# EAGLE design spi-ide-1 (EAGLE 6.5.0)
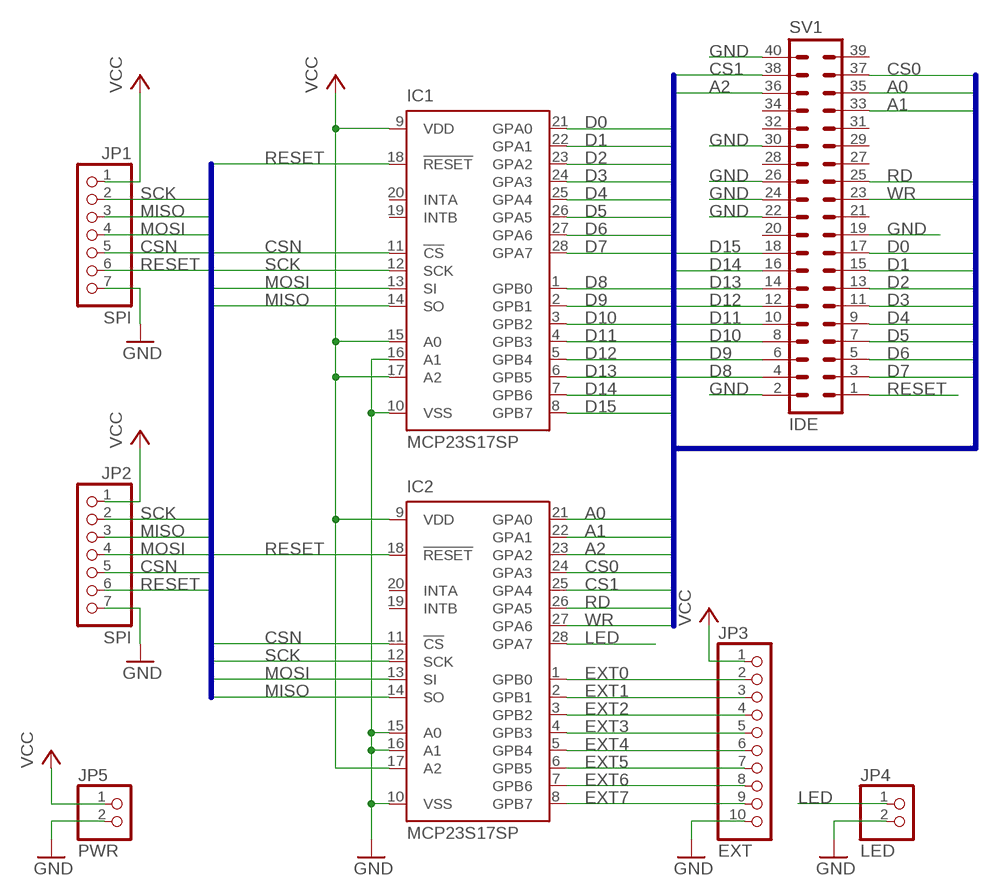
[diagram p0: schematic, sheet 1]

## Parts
IC1  MCP23S17SP  [DIL28-3]
IC2  MCP23S17SP  [DIL28-3]
JP1  SPI  PINHD-1X7  [1X07]
JP2  SPI  PINHD-1X7  [1X07]
JP3  EXT  PINHD-1X10  [1X10]
JP4  LED  PINHD-1X2  [1X02]
JP5  PWR  PINHD-1X2  [1X02]
SV1  IDE  ML40L  [ML40L]

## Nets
A0: IC2.21(GPA0) SV1.35
A1: IC2.22(GPA1) SV1.33
A2: IC2.23(GPA2) SV1.36
CS0: IC2.24(GPA3) SV1.37
CS1: IC2.25(GPA4) SV1.38
CSN: IC1.11(!CS) IC2.11(!CS) JP1.5 JP2.5
D0: IC1.21(GPA0) SV1.17
D1: IC1.22(GPA1) SV1.15
D2: IC1.23(GPA2) SV1.13
D3: IC1.24(GPA3) SV1.11
D4: IC1.25(GPA4) SV1.9
D5: IC1.26(GPA5) SV1.7
D6: IC1.27(GPA6) SV1.5
D7: IC1.28(GPA7) SV1.3
D8: IC1.1(GPB0) SV1.4
D9: IC1.2(GPB1) SV1.6
D10: IC1.3(GPB2) SV1.8
D11: IC1.4(GPB3) SV1.10
D12: IC1.5(GPB4) SV1.12
D13: IC1.6(GPB5) SV1.14
D14: IC1.7(GPB6) SV1.16
D15: IC1.8(GPB7) SV1.18
EXT0: IC2.1(GPB0) JP3.2
EXT1: IC2.2(GPB1) JP3.3
EXT2: IC2.3(GPB2) JP3.4
EXT3: IC2.4(GPB3) JP3.5
EXT4: IC2.5(GPB4) JP3.6
EXT5: IC2.6(GPB5) JP3.7
EXT6: IC2.7(GPB6) JP3.8
EXT7: IC2.8(GPB7) JP3.9
GND: IC1.10(VSS) IC1.16(A1) IC2.10(VSS) IC2.15(A0) IC2.16(A1) JP1.7 JP2.7 JP3.10 JP4.2 JP5.2 SV1.2 SV1.19 SV1.22 SV1.24 SV1.26 SV1.30 SV1.40
LED: IC2.28(GPA7) JP4.1
MISO: IC1.14(SO) IC2.14(SO) JP1.3 JP2.3
MOSI: IC1.13(SI) IC2.13(SI) JP1.4 JP2.4
RD: IC2.26(GPA5) SV1.25
RESET: IC1.18(!RESET) IC2.18(!RESET) JP1.6 JP2.6 SV1.1
SCK: IC1.12(SCK) IC2.12(SCK) JP1.2 JP2.2
VCC: IC1.9(VDD) IC1.15(A0) IC1.17(A2) IC2.9(VDD) IC2.17(A2) JP1.1 JP2.1 JP3.1 JP5.1
WR: IC2.27(GPA6) SV1.23
Unconnected: IC1.19(INTB) IC1.20(INTA) IC2.19(INTB) IC2.20(INTA) SV1.20 SV1.21 SV1.27 SV1.28 SV1.29 SV1.31 SV1.32 SV1.34 SV1.39

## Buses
BUS_SPI:SCK,MISO,MOSI,CSN,RESET
IDE:D[0..15],A[0..2],CS[0..1],RD,WR

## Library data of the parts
IC1 IC2 = microchip:MCP23S17: http://ww1.microchip.com/downloads/en/DeviceDoc/21952a.pdf Source: http://ww1.microchip.com/downloads/en/DeviceDoc/21952a.pdf; MF: MICROCHIP; MPN: MCP23S17-E/SP; OC_FARNELL: 1292238; OC_NEWARK: 31K2951
JP1 JP2 = pinhead:PINHD-1X7: PIN HEADER
JP3 = pinhead:PINHD-1X10: PIN HEADER
JP4 JP5 = pinhead:PINHD-1X2: PIN HEADER
SV1 = con-harting-ml:ML40: HARTING; OC_FARNELL: unknown; OC_NEWARK: unknown

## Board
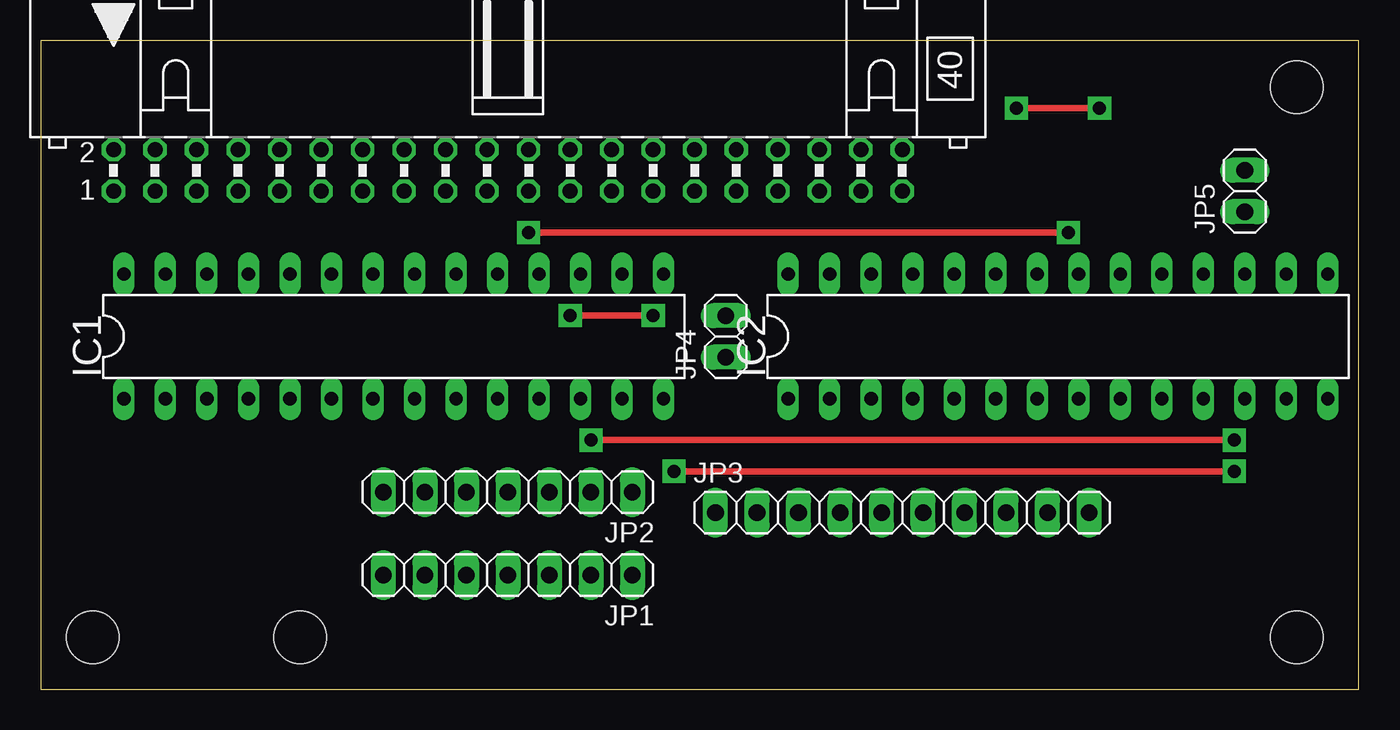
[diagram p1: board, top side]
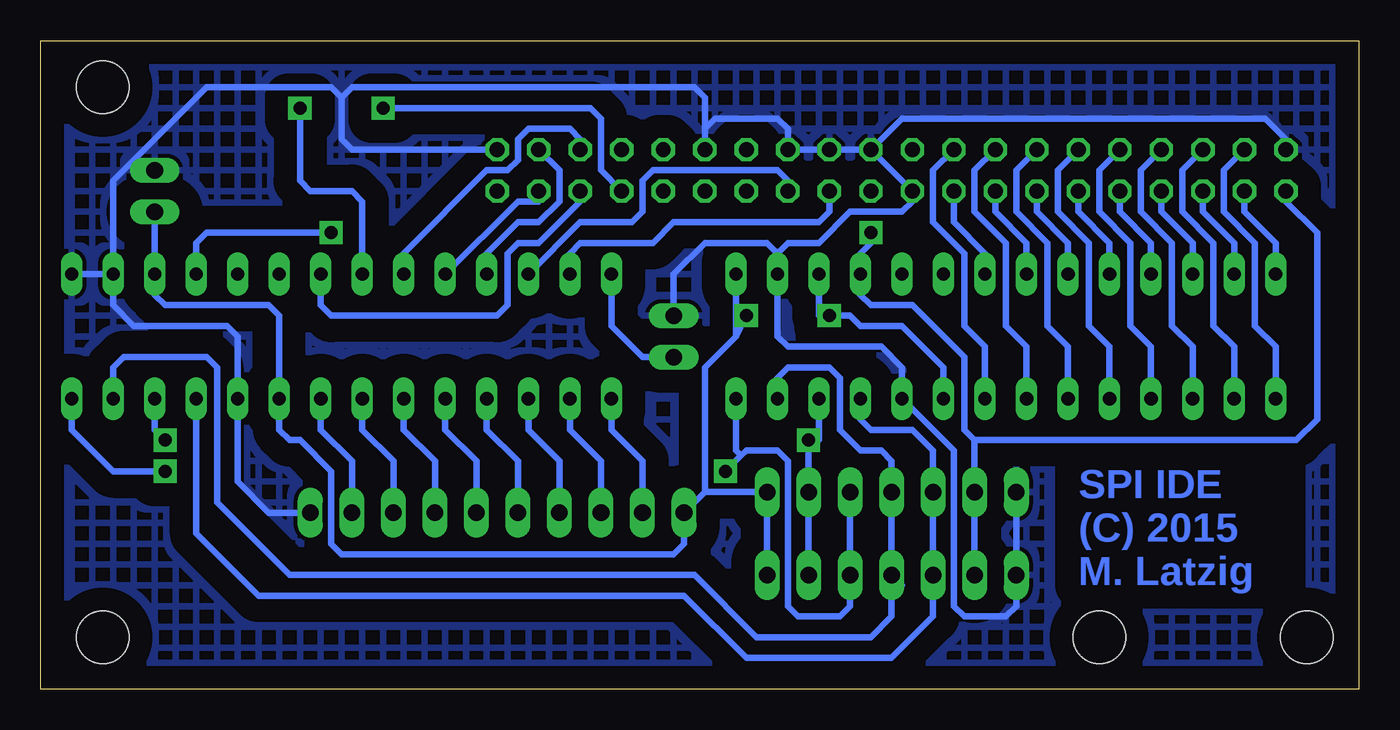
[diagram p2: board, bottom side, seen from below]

Size 80.62 x 39.67 mm. Coordinates in mm from the lower left corner, seen from the top.
Outline: 0,0 80.62,0 80.62,39.67 0,39.67 0,0
Copper layers (1*16): Top 0.035mm / dielectric 1.5mm / Bottom 0.035mm
Design rules "default": minimum track width 10mil, minimum drill 24mil, track to track 8mil, track to pad 8mil, pad to pad 8mil, via to via 8mil, smd to smd 8mil, copper to edge 40mil, drill to drill 8mil, minimum pad ring 10mil, minimum via ring 8mil, stop-mask expansion 4mil, vias tented up to drill 0mil, thermal gap 10mil
Holes 3.2 mm at 76.83,36.83 76.83,3.17 3.17,3.17 15.88,3.17

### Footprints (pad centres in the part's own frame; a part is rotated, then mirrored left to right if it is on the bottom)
DIL28-3 = drill 0.813 long: 1 -16.51,-3.81; 2 -13.97,-3.81; 3 -11.43,-3.81; 4 -8.89,-3.81; 5 -6.35,-3.81; 6 -3.81,-3.81; 7 -1.27,-3.81; 8 1.27,-3.81; 9 3.81,-3.81; 10 6.35,-3.81; 11 8.89,-3.81; 12 11.43,-3.81; 13 13.97,-3.81; 14 16.51,-3.81; 15 16.51,3.81; 16 13.97,3.81; 17 11.43,3.81; 18 8.89,3.81; 19 6.35,3.81; 20 3.81,3.81; 21 1.27,3.81; 22 -1.27,3.81; 23 -3.81,3.81; 24 -6.35,3.81; 25 -8.89,3.81; 26 -11.43,3.81; 27 -13.97,3.81; 28 -16.51,3.81
1X07 = drill 1.016 long: 1 -7.62,0; 2 -5.08,0; 3 -2.54,0; 4 0,0; 5 2.54,0; 6 5.08,0; 7 7.62,0
1X10 = drill 1.016 long: 1 -11.43,0; 2 -8.89,0; 3 -6.35,0; 4 -3.81,0; 5 -1.27,0; 6 1.27,0; 7 3.81,0; 8 6.35,0; 9 8.89,0; 10 11.43,0
1X02 = drill 1.016 long: 1 -1.27,0; 2 1.27,0
ML40L = drill 0.914 octagon: 1 -24.13,-1.27; 2 -24.13,1.27; 3 -21.59,-1.27; 4 -21.59,1.27; 5 -19.05,-1.27; 6 -19.05,1.27; 7 -16.51,-1.27; 8 -16.51,1.27; 9 -13.97,-1.27; 10 -13.97,1.27; 11 -11.43,-1.27; 12 -11.43,1.27; 13 -8.89,-1.27; 14 -8.89,1.27; 15 -6.35,-1.27; 16 -6.35,1.27; 17 -3.81,-1.27; 18 -3.81,1.27; 19 -1.27,-1.27; 20 -1.27,1.27; 21 1.27,-1.27; 22 1.27,1.27; 23 3.81,-1.27; 24 3.81,1.27; 25 6.35,-1.27; 26 6.35,1.27; 27 8.89,-1.27; 28 8.89,1.27; 29 11.43,-1.27; 30 11.43,1.27; 31 13.97,-1.27; 32 13.97,1.27; 33 16.51,-1.27; 34 16.51,1.27; 35 19.05,-1.27; 36 19.05,1.27; 37 21.59,-1.27; 38 21.59,1.27; 39 24.13,-1.27; 40 24.13,1.27

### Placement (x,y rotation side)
IC1  21.59,21.59 0 top
IC2  62.23,21.59 0 top
JP1  28.57,6.99 180 top
JP2  28.57,12.06 180 top
JP3  52.7,10.79 0 top
JP4  41.91,21.59 90 top
JP5  73.66,30.48 90 top
SV1  28.57,31.75 0 top

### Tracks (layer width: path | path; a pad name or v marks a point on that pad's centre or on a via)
A0
  Bottom 0.406: SV1.35 47.62,29.84 50.16,27.3 51.44,27.3 52.07,26.67 52.07,23.5 52.7,22.86 62.87,22.86 63.5,23.5 IC2.21
A1  (via drill 0.8 pad 1.42)
  Top 0.406: v59.69,35.56 v64.77,35.56
  Bottom 0.406: SV1.33 46.35,31.75 46.35,34.92 46.99,35.56 v59.69,35.56 | v64.77,35.56 64.77,31.11 64.14,30.48 61.59,30.48 60.96,29.84 IC2.22
A2
  Bottom 0.406: SV1.36 47.62,33.66 48.26,34.29 50.8,34.29 51.44,33.66 51.44,32.38 52.07,31.75 53.34,31.75 58.42,26.67 IC2.23
CS0
  Bottom 0.406: SV1.37 50.16,29.84 51.44,29.84 IC2.24
CS1
  Bottom 0.406: IC2.25 53.34,26.67 51.44,28.57 50.16,28.57 48.9,29.84 48.9,31.75 SV1.38
CSN
  Bottom 0.406: IC1.11 30.48,16.51 29.84,15.88 27.3,15.88 26.04,14.61 JP2.5 JP1.5 26.04,4.45 28.57,1.91 37.47,1.91 41.27,5.71 67.31,5.71 71.12,9.53 IC2.11
D0
  Bottom 0.406: IC1.21 22.86,26.67 24.77,28.57 SV1.17
D1
  Bottom 0.406: IC1.22 20.32,27.3 22.23,29.21 SV1.15
D2
  Bottom 0.406: IC1.23 17.78,27.3 19.68,29.21 SV1.13
D3
  Bottom 0.406: IC1.24 15.24,27.3 17.14,29.21 SV1.11
D4
  Bottom 0.406: IC1.25 12.7,27.3 14.61,29.21 SV1.9
D5
  Bottom 0.406: IC1.26 10.16,27.3 12.06,29.21 SV1.7
D6
  Bottom 0.406: IC1.27 7.62,27.3 9.53,29.21 SV1.5
D7
  Bottom 0.406: IC1.28 5.08,27.3 6.99,29.21 SV1.3
D8
  Bottom 0.406: IC1.1 5.08,20.95 6.35,22.23 6.35,27.3 8.26,29.21 8.26,31.75 SV1.4
D9
  Bottom 0.406: IC1.2 7.62,20.95 8.89,22.23 8.89,27.3 10.79,29.21 10.79,31.75 SV1.6
D10
  Bottom 0.406: IC1.3 10.16,20.95 11.43,22.23 11.43,27.3 13.34,29.21 13.34,31.75 SV1.8
D11
  Bottom 0.406: IC1.4 12.7,20.95 13.97,22.23 13.97,27.3 15.88,29.21 15.88,31.75 SV1.10
D12
  Bottom 0.406: IC1.5 15.24,20.95 16.51,22.23 16.51,27.3 18.41,29.21 18.41,31.75 SV1.12
D13
  Bottom 0.406: IC1.6 17.78,20.95 19.05,22.23 19.05,27.3 20.95,29.21 20.95,31.75 SV1.14
D14
  Bottom 0.406: IC1.7 20.32,20.95 21.59,22.23 21.59,27.3 23.5,29.21 23.5,31.75 SV1.16
D15
  Bottom 0.406: IC1.8 22.86,20.95 24.13,22.23 24.13,26.67 26.04,28.57 26.04,31.75 SV1.18
EXT0
  Bottom 0.406: JP3.2 43.81,13.97 45.72,15.88 IC2.1
EXT1
  Bottom 0.406: JP3.3 46.35,13.97 48.26,15.88 IC2.2
EXT2
  Bottom 0.406: JP3.4 48.9,13.97 50.8,15.88 IC2.3
EXT3
  Bottom 0.406: JP3.5 51.44,13.97 53.34,15.88 IC2.4
EXT4
  Bottom 0.406: JP3.6 53.98,13.97 55.88,15.88 IC2.5
EXT5
  Bottom 0.406: JP3.7 56.52,13.97 58.42,15.88 IC2.6
EXT6
  Bottom 0.406: JP3.8 59.05,13.97 60.96,15.88 IC2.7
EXT7
  Bottom 0.406: JP3.9 61.59,13.97 63.5,15.88 IC2.8
GND
  Bottom 0.406: SV1.2 4.45,33.66 5.71,34.92 27.94,34.92 SV1.22 | SV1.22 SV1.19 27.3,29.84 27.94,29.21 31.11,29.21 33.02,27.3 34.92,27.3 35.56,26.67 | IC2.16 76.2,23.5 74.93,22.23 69.22,22.23 68.58,21.59 IC2.10 68.58,12.7 66.67,10.79 JP3.10 | IC2.16 IC2.15 | JP2.7 JP1.7 20.95,5.08 21.59,4.45 24.13,4.45 24.77,5.08 24.77,14.61 IC1.10 27.94,19.68 29.21,20.95 34.92,20.95 35.56,21.59 IC1.16 35.56,26.67 | SV1.40 61.59,33.02 62.23,33.66 62.23,36.2 | 62.23,36.2 61.59,36.83 40.64,36.83 40.01,36.2 40.01,34.29 | 40.01,34.29 SV1.30 | 40.01,34.29 39.37,34.92 35.56,34.92 34.92,34.29 SV1.26 SV1.24 SV1.22 | JP4.2 41.91,25.4 40.01,27.3 36.2,27.3 35.56,26.67 | IC2.16 76.2,31.11 70.48,36.83 62.87,36.83 62.23,36.2
  pour Bottom (isolate 1.422, hatched): 0,40.01 80.64,40.01 80.64,0 0,0
LED
  Bottom 0.406: JP4.1 43.81,20.32 45.72,22.23 IC2.28
MISO  (via drill 0.8 pad 1.42)
  Top 0.406: v73.03,13.34 v38.73,13.34
  Bottom 0.406: JP2.3 JP1.3 31.11,5.08 31.75,4.45 34.29,4.45 34.92,5.08 34.92,13.97 35.56,14.61 37.47,14.61 37.78,14.29 | 37.78,14.29 38.1,14.61 IC1.14 | IC2.14 78.74,15.88 76.2,13.34 v73.03,13.34 | v38.73,13.34 37.78,14.29
MOSI
  Bottom 0.406: JP1.4 JP2.4 28.57,13.97 29.21,14.61 30.48,14.61 31.75,15.88 31.75,19.05 32.38,19.68 34.92,19.68 35.56,19.05 IC1.13 | JP1.4 27.94,6.35 | IC2.13 76.2,19.68 75.56,20.32 70.48,20.32 69.85,19.68 69.85,11.43 65.41,6.99 40.64,6.99 36.83,3.17 29.84,3.17 28.57,4.45 JP1.4
RD
  Bottom 0.406: IC2.26 47.62,28.57 44.45,28.57 43.81,29.21 43.81,31.11 43.18,31.75 35.56,31.75 34.92,31.11 SV1.25
RESET  (via drill 0.8 pad 1.42)
  Top 0.406: v29.84,27.94 v62.87,27.94
  Bottom 0.406: JP1.6 JP2.6 23.5,15.24 | 23.5,15.24 24.13,15.88 24.13,20.32 27.3,23.5 29.84,23.5 30.48,24.13 IC1.18 30.48,26.67 29.84,27.3 v29.84,27.94 | SV1.1 4.45,29.84 2.54,27.94 2.54,16.51 3.81,15.24 23.5,15.24 | v62.87,27.94 70.48,27.94 71.12,27.3 IC2.18
SCK  (via drill 0.8 pad 1.42)
  Top 0.406: v73.03,15.24 v33.66,15.24
  Bottom 0.406: JP1.2 JP2.2 33.66,14.61 33.34,14.92 | 33.34,14.92 33.02,15.24 IC1.12 | IC2.12 73.66,15.88 v73.03,15.24 | v33.66,15.24 33.34,14.92
VCC  (via drill 0.8 pad 1.42)
  Top 0.406: v37.47,22.86 v32.38,22.86
  Bottom 0.406: 40.01,12.06 JP3.1 41.27,8.89 41.91,8.26 62.23,8.26 62.87,8.89 62.87,13.34 64.77,15.24 65.41,15.24 66.04,15.88 IC2.9 66.04,22.86 66.67,23.5 73.03,23.5 73.66,24.13 IC2.17 JP5.1 | 40.01,12.06 JP2.1 JP1.1 | IC1.9 25.4,19.68 27.94,22.23 30.48,22.23 31.11,22.86 v32.38,22.86 33.02,22.86 IC1.17 | IC1.15 38.1,21.59 | 38.1,21.59 40.01,19.68 40.01,12.06 | 38.1,21.59 v37.47,22.86
WR
  Bottom 0.406: IC2.27 48.26,26.67 47.62,27.3 43.18,27.3 41.91,28.57 33.02,28.57 32.38,29.21 SV1.23

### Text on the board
Bottom: SPI IDE / (C) 2015 / M. Latzig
